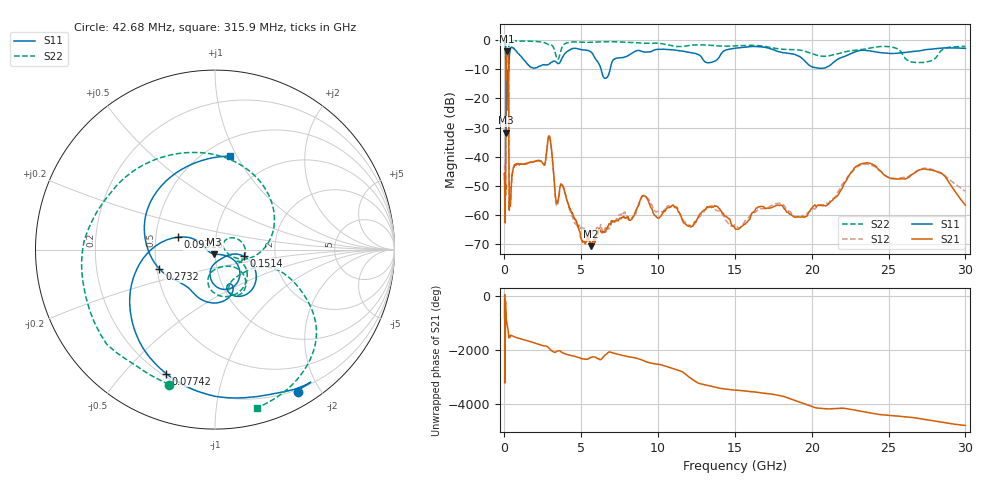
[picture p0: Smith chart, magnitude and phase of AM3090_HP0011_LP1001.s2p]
! Date/Time: Thu, Feb 28, 2019 1:56 PM
! Network Analyzer: Agilent Technologies E8364B Rev: A.07.50.67
! Sweep from 0.010 to 30.000 GHz, 1601 Points, Sweep Type: LOG
! Power Supply: 5.023 V, 0.002 A
# Hz S DB R 50
!freq MagS11 AngS11 MagS21 AngS21 MagS12 AngS12 MagS22 AngS22
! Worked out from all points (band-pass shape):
!   1601 points, 10 MHz to 30 GHz, reference 50 ohm
!   highest |S21| = -3.88 dB at 152.9 MHz (marker M1); lowest = -70.7 dB at 5.64 GHz (marker M2)
!   |S21| within 3 dB of the highest: 102.7 MHz to 249.1 MHz (146.4 MHz wide, 83.2 % of centre)
!   lowest |S11| = -31.8 dB at 100.9 MHz (marker M3), VSWR 1.05, Z = 49.5 - j2.51 ohm
!   |S11| at or under -10 dB: 91.54 MHz to 271.4 MHz (179.9 MHz wide, 99.1 % of centre); 6.288 GHz to 6.877 GHz (588.5 MHz wide, 8.94 % of centre)
!   |S22| runs from -26.3 to -0.1 dB; largest |S21 - S12| = 0.01
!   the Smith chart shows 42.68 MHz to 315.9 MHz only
!   S11 on the Smith chart (normalised r, x): 42.68 MHz: 0.17, -1.73; 77.42 MHz: 0.21, -0.66; 93.16 MHz: 0.65, +0.09; 151.4 MHz: 1.37, -0.10; 273.2 MHz: 0.52, -0.13; 315.9 MHz: 0.65, +0.94
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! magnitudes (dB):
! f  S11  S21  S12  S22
! 10 MHz  -0.2  -45.7  -42.9  -0.7
! 38.04 MHz  -0.5  -61.0  -59.6  -1.6
! 42.68 MHz  -0.8  -62.5  -61.4  -2.0
! 47.65 MHz  -0.8  -49.5  -52.0  -2.0
! 77.42 MHz  -2.6  -44.6  -46.2  -4.7
! 93.16 MHz  -13.2  -14.3  -14.2  -12.3
! 100.9 MHz  -31.8  -7.5  -7.5  -25.6
! 116.7 MHz  -12.9  -5.0  -5.0  -17.0
! 144.7 MHz  -22.0  -3.9  -3.9  -17.0
! 151.4 MHz  -15.8  -3.9  -3.8  -15.5
! 152.9 MHz  -14.8  -3.9  -3.8  -15.1
! 273.2 MHz  -9.7  -16.3  -16.3  -7.9
! 315.9 MHz  -5.6  -58.4  -54.4  -0.8
! 550.5 MHz  -2.7  -44.5  -44.2  -0.2
! 2.084 GHz  -9.5  -41.4  -41.4  -0.5
! 2.928 GHz  -8.1  -33.0  -33.0  -1.6
! 3.402 GHz  -7.7  -56.0  -57.0  -6.3
! 5.64 GHz  -4.1  -70.7  -66.4  -0.8
! 7.926 GHz  -5.6  -61.0  -60.1  -0.8
! 19.12 GHz  -5.4  -60.6  -60.4  -3.4
! 23.48 GHz  -3.5  -42.2  -42.6  -3.0
! 30 GHz  -2.8  -56.6  -51.9  -2.2
